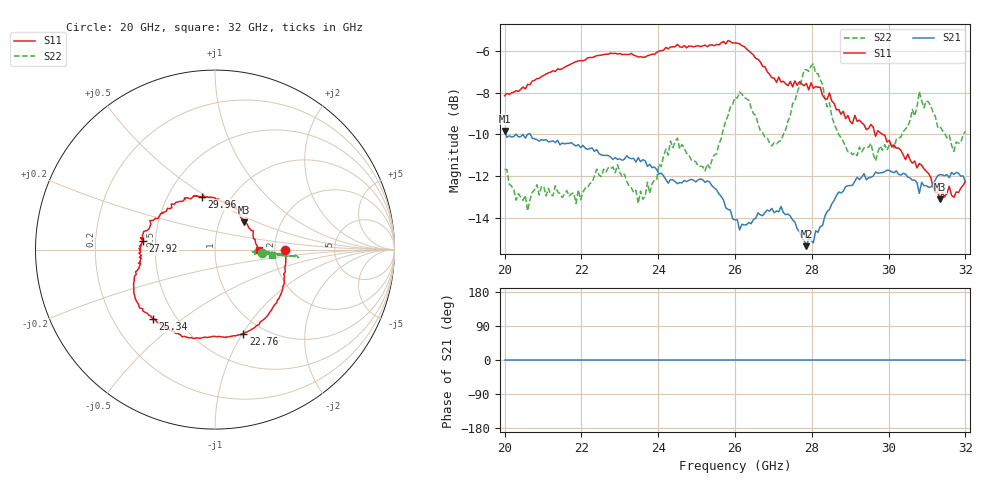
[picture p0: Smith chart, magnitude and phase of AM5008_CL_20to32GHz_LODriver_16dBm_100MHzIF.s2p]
!Keysight Technologies,N5245B,MY58422270,A.16.20.02
!Mixer S2P File: Scalar Mixer Measurement
!Calibration State: On
!Parameters: Stimulus Freq, S11, SC21, SC12, S22
# Hz  S  DB  R  50.0
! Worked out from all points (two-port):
!   201 points, 20 GHz to 32 GHz, reference 50 ohm
!   highest |S21| = -9.84 dB at 20 GHz (marker M1); lowest = -15.4 dB at 27.86 GHz (marker M2)
!   |S21| within 3 dB of the highest: start of sweep to 25.58 GHz; 28.67 GHz to end of sweep
!   lowest |S11| = -13.1 dB at 31.34 GHz (marker M3), VSWR 1.57, Z = 65.3 + j20.9 ohm
!   |S11| at or under -10 dB: 29.64721 GHz to 29.68027 GHz (33.07 MHz wide, 0.111 % of centre); 29.84 GHz to end of sweep
!   |S22| runs from -13.7 to -6.6 dB; largest |S21 - S12| = 0.32
!   S11 on the Smith chart (normalised r, x): 20 GHz: 2.29, -0.01; 22.76 GHz: 0.81, -1.01; 25.34 GHz: 0.37, -0.39; 27.92 GHz: 0.43, +0.05; 29.96 GHz: 0.73, +0.48; 32 GHz: 1.65, -0.00
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2e10  -8.15 -0.3  -9.84 0.0  -200.00 90.0  -11.67 -4.7
2.06e10  -7.60 -21.4  -9.99 0.0  -200.00 90.0  -13.66 -3.3
2.084e10  -7.33 -26.4  -10.25 0.0  -200.00 90.0  -12.41 -1.9
2.204e10  -6.47 -56.7  -10.53 0.0  -200.00 90.0  -12.78 -4.8
2.276e10  -6.10 -71.4  -11.09 0.0  -200.00 90.0  -11.65 -5.5
2.348e10  -6.30 -87.3  -11.11 0.0  -200.00 90.0  -13.31 -1.9
2.402e10  -6.01 -99.4  -11.90 0.0  -200.00 90.0  -11.42 -3.6
2.45e10  -5.69 -110.5  -12.36 0.0  -200.00 90.0  -10.18 -4.3
2.534e10  -5.72 -131.9  -12.29 0.0  -200.00 90.0  -11.62 -3.3
2.6e10  -5.62 -145.6  -14.10 0.0  -200.00 90.0  -8.23 -4.5
2.696e10  -7.29 -167.1  -13.55 0.0  -200.00 90.0  -10.56 -2.1
2.786e10  -7.56 177.7  -15.36 0.0  -200.00 90.0  -6.90 -4.4
2.792e10  -7.87 173.3  -14.98 0.0  -200.00 90.0  -6.98 -4.0
2.804e10  -7.79 171.6  -15.20 0.0  -200.00 90.0  -6.62 -5.5
2.894e10  -9.10 139.0  -12.46 0.0  -200.00 90.0  -10.83 -3.8
2.996e10  -10.37 103.9  -11.71 0.0  -200.00 90.0  -10.76 -4.5
3.002e10  -10.29 101.9  -11.73 0.0  -200.00 90.0  -10.50 -3.6
3.068e10  -11.28 77.4  -12.19 0.0  -200.00 90.0  -9.12 -3.8
3.08e10  -11.40 74.1  -12.83 0.0  -200.00 90.0  -7.95 -4.6
3.134e10  -13.11 43.5  -11.93 0.0  -200.00 90.0  -9.62 -3.8
3.17e10  -13.01 15.4  -11.93 0.0  -200.00 90.0  -10.81 -4.3
3.2e10  -12.25 -0.2  -12.27 0.0  -200.00 90.0  -9.86 -5.6
